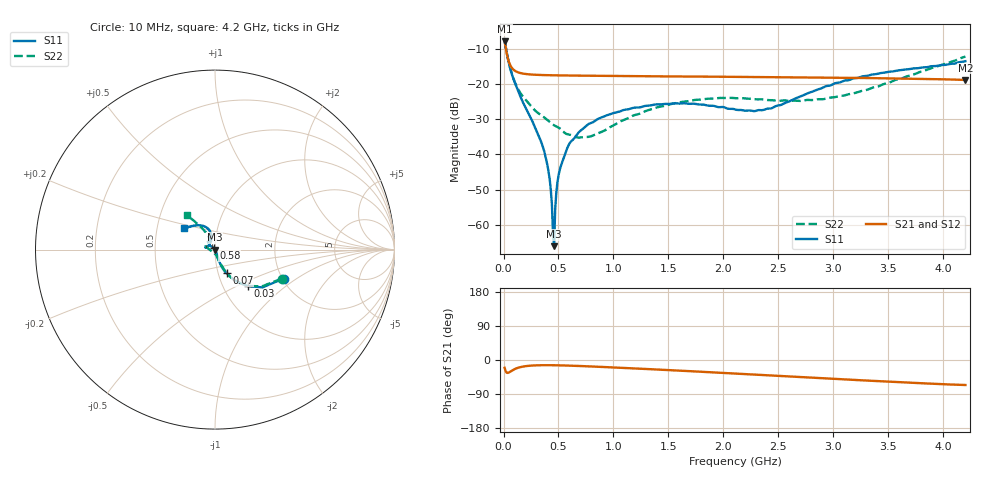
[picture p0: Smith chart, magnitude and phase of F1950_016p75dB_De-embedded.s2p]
! Integrated Device Technology
! Corporate Headquarters
! 6024 Silver Creek Valley Road
! San Jose, CA 95138  USA
! Phone:  1-408-284-8200
! Toll Free:  1-800-223-1366
! Webpage:  http://www.idt.com/
! Timing and RF Division
! 515 Groton Road, Suite 102
! Westford, MA 01886-6024
! Device:  F1950
! Description: 7-bit 0.25 dB Digital Step Attenuator
! Frequency:  150.0 -  4000.00 MHz
! Package:  4x4 mm Thin QFN Plastic Package: 24 pin
! Ports:  2 RF, 12 DC
!  Pin  1  = D0
!  Pin  2  = VDD
!  Pin  3  = Vmode
!  Pin  4  = GND
!  Pin  5  = RF1  =  Port 1
!  Pin  6  = GND
!  Pin  7  = GND
!  Pin  8  = GND
!  Pin  9  = GND
!  Pin 10  = GND
!  Pin 11  = GND
!  Pin 12  = GND
!  Pin 13  = GND
!  Pin 14  = RF2  =  Port 2
!  Pin 15  = GND
!  Pin 16  = LE
!  Pin 17  = CLK
!  Pin 18  = DATE
!  Pin 19  = D6
!  Pin 20  = D5
!  Pin 21  = D4
!  Pin 22  = D3
!  Pin 23  = D2
!  Pin 24  = D1
! State:  67
! Atten State:  16.75 dB
! Voltage:  +5.00 Volts
! Current:  Not Measured mA
! Data:  The device was measured on a the F195X evaluation board which has
!  individual transmission lines to the RF pins.  Data was collected
!  using a calibrated network analyzer.  The evaluation board was
!  de-embedded using a TRL calibration technique.
!  The reference plane is the edge of the package pin.
! Misc:  Board 2019
!  Action Tracker AT0250
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# GHz S dB R 50
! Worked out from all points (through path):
!   420 points, 10 MHz to 4.2 GHz, reference 50 ohm
!   highest |S21| = -7.84 dB at 10 MHz (marker M1); lowest = -18.8 dB at 4.2 GHz (marker M2)
!   group delay of S21, straight-line fit = 36.9 ps
!   lowest |S11| = -66.0 dB at 460 MHz (marker M3), VSWR 1.00, Z = 50 + j0.0355 ohm
!   |S11| at or under -10 dB: 23.24 MHz to end of sweep
!   |S22| runs from -35.2 to -7.8 dB; largest |S21 - S12| = 0.0002
!   S11 on the Smith chart (normalised r, x): 10 MHz: 2.03, -0.79; 30 MHz: 1.31, -0.58; 70 MHz: 1.10, -0.30; 580 MHz: 0.98, +0.02; 4.2 GHz: 0.69, +0.17
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0.01  -7.64 -22.9  -7.84 -20.6  -7.84 -20.6  -7.84 -23.5
0.03  -11.22 -47.8  -11.43 -33.8  -11.43 -33.8  -11.28 -47.7
0.07  -16.63 -64.0  -15.15 -29.2  -15.15 -29.2  -16.45 -63.3
0.16  -24.03 -70.0  -16.94 -18.3  -16.94 -18.3  -22.84 -70.9
0.36  -38.05 -62.7  -17.46 -13.7  -17.46 -13.7  -29.23 -78.4
0.41  -44.97 -64.3  -17.50 -13.7  -17.50 -13.7  -30.52 -79.7
0.42  -47.05 -65.3  -17.51 -13.7  -17.51 -13.7  -30.78 -80.6
0.44  -54.14 -67.3  -17.52 -13.8  -17.52 -13.8  -31.31 -83.0
0.46  -66.03 134.7  -17.53 -13.8  -17.53 -13.9  -31.73 -85.9
0.47  -55.51 122.1  -17.54 -13.9  -17.54 -13.9  -31.89 -87.3
0.49  -47.95 124.2  -17.55 -14.0  -17.55 -14.0  -32.19 -89.5
0.51  -44.53 127.3  -17.56 -14.1  -17.56 -14.1  -32.56 -90.7
0.58  -38.18 128.9  -17.59 -14.7  -17.59 -14.7  -34.27 -101.4
0.71  -33.02 134.9  -17.63 -16.0  -17.63 -16.0  -35.13 -125.6
0.99  -28.37 146.1  -17.72 -19.5  -17.72 -19.5  -31.90 -171.4
1.41  -25.81 162.7  -17.82 -25.4  -17.82 -25.4  -26.53 166.3
1.73  -25.59 168.4  -17.89 -30.0  -17.89 -30.0  -24.57 157.6
2.11  -27.27 158.0  -17.97 -35.9  -17.97 -35.9  -24.03 148.2
2.43  -26.94 125.7  -18.05 -40.6  -18.05 -40.6  -24.57 138.3
2.81  -22.15 104.7  -18.14 -46.6  -18.13 -46.7  -24.56 123.3
3.51  -16.51 117.2  -18.38 -57.3  -18.38 -57.3  -19.60 117.8
4.2  -13.53 146.0  -18.85 -66.0  -18.85 -66.1  -12.20 129.0
